(* Logix 5000 DataType export Banner_S15C_B21_VSC_v4; software revision 33.00 *)

TYPE Banner_S15C_B21_VSC_v4 :   // Vendor Specific Configuration Parameter Data for S15C-B21 unit.
STRUCT
   PDI1_Metric_Selection : SINT;   // 0 = Disabled, 1 = Count, 2 = Duration, 3 = Events per Minute
   PDI1_Port_Selection : SINT;   // 0 = Port 1
   PDI1_Channel_Selection : SINT;   // 0 = Discrete 1, 1 = Discrete 2
   PDI2_Metric_Selection : SINT;   // 0 = Disabled, 1 = Count, 2 = Duration, 3 = Events per Minute
   PDI2_Port_Selection : SINT;   // 0 = Port 1
   PDI2_Channel_Selection : SINT;   // 0 = Discrete 1, 1 = Discrete 2
   PDI3_Metric_Selection : SINT;   // 0 = Disabled, 1 = Count, 2 = Duration, 3 = Events per Minute
   PDI3_Port_Selection : SINT;   // 0 = Port 1
   PDI3_Channel_Selection : SINT;   // 0 = Discrete 1, 1 = Discrete 2
   PDI4_Metric_Selection : SINT;   // 0 = Disabled, 1 = Count, 2 = Duration, 3 = Events per Minute
   PDI4_Port_Selection : SINT;   // 0 = Port 1
   PDI4_Channel_Selection : SINT;   // 0 = Discrete 1, 1 = Discrete 2
END_STRUCT
END_TYPE
